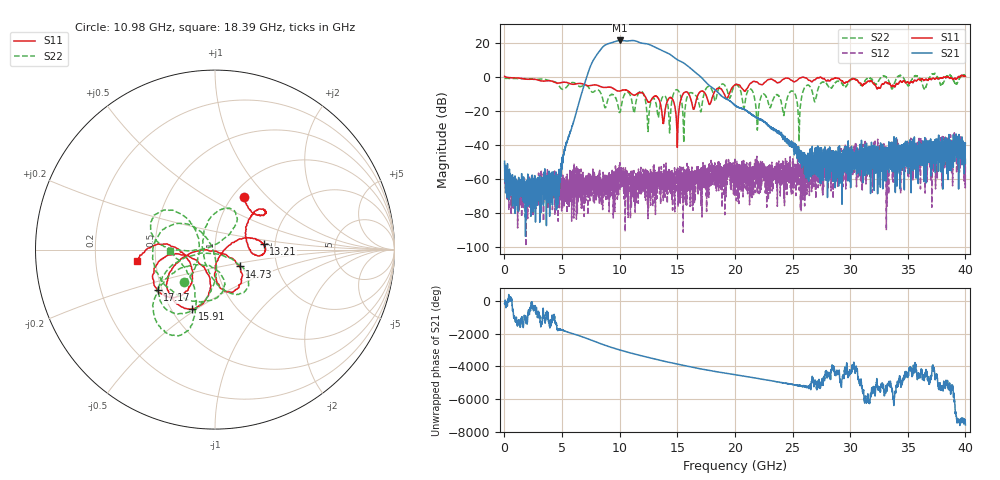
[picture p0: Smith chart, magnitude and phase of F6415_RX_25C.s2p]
!Keysight Technologies,N5245B,MY52451815,A.15.70.20
!Date: Wednesday, April 17, 2024 14:30:00
!Correction: S33(C  2-Port  )
!S43(C  2-Port  )
!S34(C  2-Port  )
!S44(C  2-Port  )
!S2P File: Measurements: S33, S43, S34, S44:
# Hz S  RI  R 50
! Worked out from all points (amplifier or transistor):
!   4000 points, 10 MHz to 40 GHz, reference 50 ohm
!   highest |S21| = 21.7 dB at 10.05 GHz (marker M1)
!   |S21| within 3 dB of that: 8.674 GHz to 12.77 GHz (4.097 GHz wide, 38.2 % of centre)
!   unconditionally stable (mu >= 1): 149.6 MHz to 25.85 GHz; 25.98 GHz to 27.43 GHz; 27.45 GHz to 32.69 GHz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
!   at 6.67 GHz: K = 4764.54, MAG = -6.2 dB, |S12| = -77.2 dB
!   at 20.01 GHz: K = 659.01, MAG = -12.9 dB, |S12| = -53.1 dB
!   at 40 GHz: K = 416.16, MSG = 4.2 dB, |S12| = -47.4 dB
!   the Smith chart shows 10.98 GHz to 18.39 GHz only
!   S11 on the Smith chart (normalised r, x): 10.98 GHz: 1.12, +0.74; 13.21 GHz: 1.74, +0.12; 14.73 GHz: 1.29, -0.25; 15.91 GHz: 0.64, -0.48; 17.17 GHz: 0.47, -0.25; 18.39 GHz: 0.39, -0.06
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1e7  1.037 0.2047  -0.00201 -0.00266  0.0024 0.00172  -0.9252 0.0149
6.68e9  -0.5487 0.3435  0.3196 -0.0297  0.00025 -0.000398  0.5358 0.0306
8.43e9  -0.1409 0.4958  -2.058 -6.825  0.000294 0.000404  0.0747 -0.2862
8.78e9  -0.0367 0.4976  -8.749 2.253  -0.000158 -0.000301  -0.0872 -0.094
9.13e9  0.0214 0.508  1.419 9.908  0.00126 -0.000532  -0.247 -0.1357
9.56e9  0.0574 0.4362  10.71 -2.829  2.84e-05 0.000395  -0.1291 -0.2443
1.005e10  0.1605 0.3606  -5.642 -10.7  0.000401 -0.000701  -0.0916 -0.0389
1.045e10  0.1863 0.3793  -11.26 3.45  0.00136 0.000161  -0.3227 -0.0572
1.098e10  0.1594 0.2916  6.062 10.3  -5.42e-05 -0.000825  -0.1732 -0.1824
1.132e10  0.2196 0.1984  11.8 -1.191  -0.000696 -0.000562  -0.0923 0.0653
1.174e10  0.2824 0.2136  1.894 -10.3  0.000437 -0.000303  -0.3178 0.2035
1.232e10  0.1783 0.1423  -9.651 0.502  0.00032 0.000874  -0.1298 -0.00559
1.321e10  0.2709 0.0316  6.361 3.547  0.000387 0.000357  -0.055 0.1198
1.334e10  0.2323 0.0527  6.892 0.8981  -0.000261 -0.0016  -0.067 -0.00245
1.473e10  0.1368 -0.0939  -3.206 2.009  0.00122 -2.35e-05  -0.3084 -0.192
1.591e10  -0.1256 -0.3293  1.894 -0.9829  0.000988 0.000295  -0.2661 0.126
1.717e10  -0.3201 -0.2255  -0.8342 0.3924  0.00159 0.000103  -0.1522 -0.0939
1.839e10  -0.4352 -0.0613  0.3925 0.00957  -0.000907 0.00174  -0.2516 -0.00812
2.001e10  -0.5908 -0.1167  -0.1484 0.00157  -0.0022 0.000167  -0.469 0.3195
2.667e10  -0.5648 0.4696  -0.00336 0.000533  -0.0029 -0.00195  0.3559 -0.2045
3.334e10  0.6556 -0.0302  0.000815 0.00131  -4.51e-06 -0.00036  -0.2642 -0.7511
4e10  -0.756 -0.734  0.0104 -0.00422  -0.00333 -0.00267  -1.163 -0.0888
